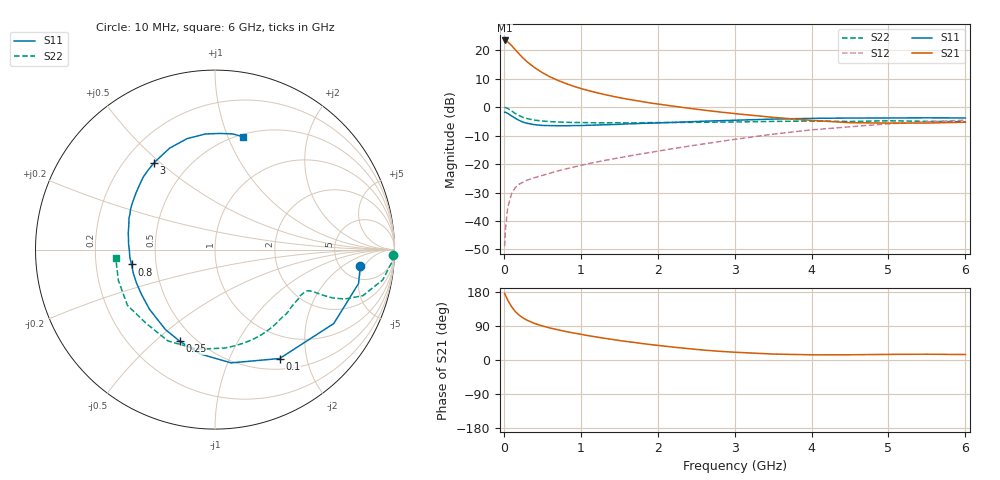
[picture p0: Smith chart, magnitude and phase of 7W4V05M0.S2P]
! Infineon Technologies  Discrete & RF Semiconductors
! BFS17W
! Si NPN RF Bipolar Junction Transistor in SOT323
! VCE = 4 V  IC = 5 mA
! Common Emitter S-Parameters:  August  1999
# GHz  S  MA  R  50
!  f  S11  S21  S12  S22
! GHz  MAG  ANG  MAG  ANG  MAG  ANG  MAG  ANG
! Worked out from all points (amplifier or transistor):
!   36 points, 10 MHz to 6 GHz, reference 50 ohm
!   highest |S21| = 23.5 dB at 10 MHz (marker M1)
!   |S21| within 3 dB of that: start of sweep to 140.4 MHz
!   unconditionally stable (mu >= 1): 560 MHz to 2.682 GHz; 4.396 GHz to end of sweep
!   at 250 MHz: K = 0.59, MSG = 21.8 dB, |S12| = -26.4 dB
!   at 1.4 GHz: K = 1.24, MAG = 8.2 dB, |S12| = -18.3 dB
!   at 6 GHz: K = 1.07, MAG = -2.0 dB, |S12| = -4.5 dB
!   S11 on the Smith chart (normalised r, x): 10 MHz: 7.50, -4.11; 100 MHz: 0.65, -1.56; 250 MHz: 0.41, -0.60; 800 MHz: 0.36, -0.08; 3 GHz: 0.32, +0.48; 6 GHz: 0.52, +1.14
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0.01  0.8146 -6.5  14.97 176.0  0.0036 85.7  0.9948 -1.7
0.02  0.8218 -13.3  14.97 171.0  0.0069 82.2  0.9862 -4.3
0.05  0.7795 -31.9  14.15 158.3  0.0171 75.5  0.95 -10.2
0.1  0.7057 -59.3  12.22 140.9  0.0302 63.3  0.8632 -17.3
0.15  0.6375 -81.9  10.24 127.6  0.039 55.4  0.7746 -20.8
0.2  0.5874 -98.0  8.623 118.2  0.0445 52.2  0.7112 -22.3
0.25  0.5469 -111.1  7.33 111.0  0.0481 49.0  0.6639 -22.8
0.3  0.5241 -121.8  6.35 105.2  0.0521 48.9  0.6339 -23.0
0.4  0.4938 -137.6  4.97 96.4  0.0578 49.1  0.5929 -23.2
0.5  0.4795 -148.8  4.068 89.9  0.0633 51.0  0.5727 -23.6
0.6  0.4754 -157.3  3.43 84.5  0.0693 52.6  0.559 -24.4
0.8  0.472 -169.9  2.637 75.4  0.0819 55.7  0.5443 -27.3
0.9  0.4765 -174.8  2.359 71.5  0.0883 57.5  0.5391 -28.9
1.1  0.4825 176.3  1.964 64.1  0.102 59.7  0.5355 -32.9
1.3  0.4923 169.0  1.686 57.6  0.1155 61.7  0.5322 -37.6
1.6  0.5105 159.9  1.394 48.7  0.1366 64.0  0.5314 -44.8
2.2  0.5415 144.4  1.046 34.0  0.1872 66.6  0.5403 -61.0
3  0.5914 125.0  0.774 20.5  0.2725 65.4  0.551 -84.3
3.5  0.6192 114.1  0.664 15.7  0.3366 61.9  0.564 -100.1
4.5  0.6463 94.9  0.535 13.8  0.4537 50.0  0.562 -133.0
5.5  0.652 81.2  0.528 15.2  0.5548 37.2  0.5651 -162.3
6  0.648 76.0  0.546 14.5  0.594 31.0  0.555 -175.2
